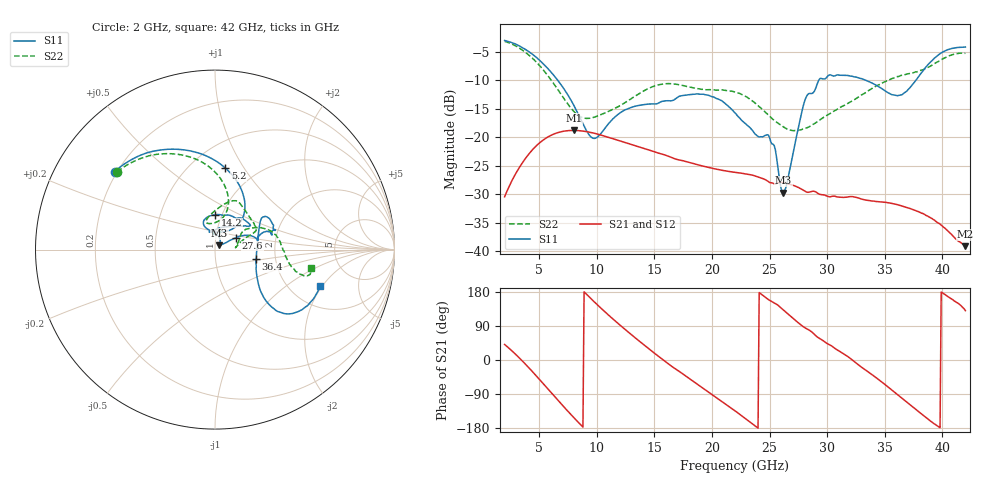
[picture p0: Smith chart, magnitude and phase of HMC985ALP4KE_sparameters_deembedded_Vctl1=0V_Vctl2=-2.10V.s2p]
!s2p File: Measurements: S11, S21, S12, S22
# GHz S dB R 50.0
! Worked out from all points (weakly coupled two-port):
!   401 points, 2 GHz to 42 GHz, reference 50 ohm
!   highest |S21| = -18.78 dB at 8 GHz (marker M1); lowest = -39.1 dB at 42 GHz (marker M2)
!   lowest |S11| = -29.7 dB at 26.2 GHz (marker M3), VSWR 1.07, Z = 52.3 + j2.41 ohm
!   |S11| at or under -10 dB: 6.618 GHz to 29.27 GHz (22.65 GHz wide, 126 % of centre); 33.37 GHz to 37.7 GHz (4.331 GHz wide, 12.2 % of centre)
!   |S22| runs from -18.8 to -3.1 dB; largest |S21 - S12| = 0.00018
!   S11 on the Smith chart (normalised r, x): 2 GHz: 0.19, +0.33; 5.2 GHz: 0.72, +0.83; 14.2 GHz: 0.93, +0.38; 27.6 GHz: 1.25, +0.17; 36.4 GHz: 1.58, -0.18; 42 GHz: 2.90, -1.91
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2  -2.99 142.2  -30.44 41.0  -30.44 41.0  -3.15 141.5
3.6  -4.32 113.1  -24.30 -4.4  -24.31 -4.4  -4.78 112.7
5.2  -6.79 82.7  -20.70 -57.3  -20.70 -57.3  -7.79 86.9
8  -14.35 47.3  -18.78 -151.8  -18.79 -151.8  -15.44 79.7
8.7  -17.23 52.2  -18.88 -173.9  -18.88 -173.9  -16.50 90.5
9.9  -20.14 89.2  -19.34 150.1  -19.35 150.0  -16.38 105.6
12.1  -15.60 112.9  -20.67 89.9  -20.68 89.9  -14.33 98.8
14.2  -14.22 89.8  -22.00 37.3  -22.00 37.3  -11.71 78.2
15.4  -13.94 73.2  -22.79 9.0  -22.79 8.9  -10.76 70.0
19.3  -12.45 34.3  -25.09 -76.0  -25.09 -76.0  -11.56 41.4
22  -15.71 52.3  -26.14 -134.1  -26.14 -134.1  -12.05 24.6
25  -20.05 98.6  -27.91 157.7  -27.92 157.6  -16.30 17.2
26.2  -29.70 44.6  -27.98 131.9  -27.99 131.9  -18.18 8.9
27.6  -17.39 29.7  -28.91 95.6  -28.91 95.7  -18.71 6.1
28.1  -13.31 20.9  -29.48 84.5  -29.49 84.5  -18.45 8.8
28.7  -12.28 13.0  -29.48 73.1  -29.48 73.0  -17.83 13.6
31  -9.06 23.3  -30.49 24.3  -30.49 24.3  -14.89 32.7
33.3  -9.94 34.2  -30.99 -25.7  -31.01 -25.7  -12.20 29.5
35.4  -12.27 12.1  -31.51 -74.0  -31.53 -74.0  -9.90 19.7
36.4  -12.58 -13.1  -31.99 -98.5  -32.00 -98.5  -9.14 13.5
39.5  -5.81 -43.4  -34.85 -172.5  -34.84 -172.4  -6.83 -14.0
42  -4.14 -19.0  -39.10 130.2  -39.08 130.1  -5.24 -11.0
